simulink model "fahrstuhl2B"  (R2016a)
settings: Solver=ode45  StartTime=0.0  StopTime=Inf  FixedStep=1e-5  MaxStep=1e-4  RelTol=1e-3
undefined symbols (not defined in the file or in its folder): s0, tS, vF
libraries: simulink x3

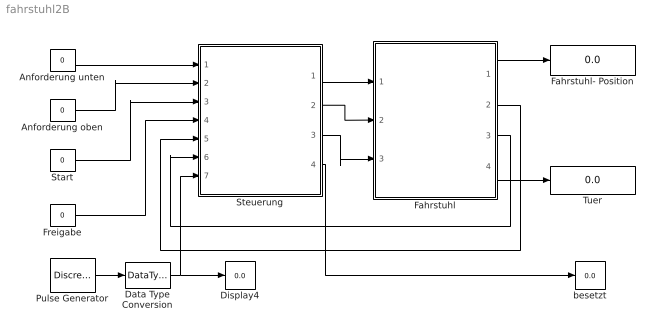
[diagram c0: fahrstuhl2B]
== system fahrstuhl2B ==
  Anforderung oben : Constant  Value=0  OutDataTypeStr=boolean
  Anforderung unten : Constant  Value=0  OutDataTypeStr=boolean
  Data Type Conversion : DataTypeConversion  OutDataTypeStr=boolean
  Display4 : Display
  Fahrstuhl : Subsystem
  Fahrstuhl- Position : Display
  Freigabe : Constant  Value=0  OutDataTypeStr=boolean
  Pulse Generator : DiscretePulseGenerator  PulseType=Time based  PulseWidth=50
  Start : Constant  Value=0  OutDataTypeStr=boolean
  Steuerung : Subsystem
  Tuer : Display
  besetzt : Display
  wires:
  Pulse Generator/1 -> Data Type Conversion/1
  Freigabe/1 -> Steuerung/4(F)
  Start/1 -> Steuerung/3(S)
  Anforderung oben/1 -> Steuerung/2(A2)
  Anforderung unten/1 -> Steuerung/1(A1)
  Fahrstuhl/1(z) -> Fahrstuhl- Position/1
  Steuerung/1(Mh) -> Fahrstuhl/1(Mh)
  Steuerung/2(Mr) -> Fahrstuhl/2(Mr)
  Steuerung/3(T) -> Fahrstuhl/3(Ti)
  Steuerung/4(Z) -> besetzt/1
  Fahrstuhl/4(T) -> Tuer/1
  Fahrstuhl/3(P2) -> Steuerung/6(P2)
  Fahrstuhl/2(P1) -> Steuerung/5(P1)
  Data Type Conversion/1 -> Steuerung/7(Takt), Display4/1

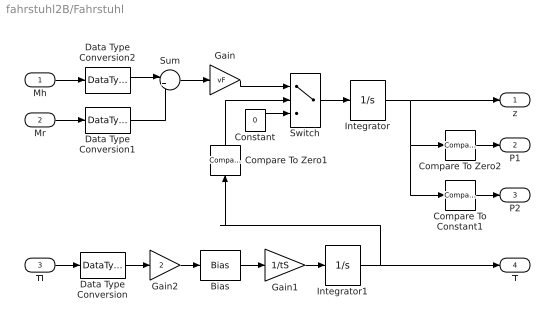
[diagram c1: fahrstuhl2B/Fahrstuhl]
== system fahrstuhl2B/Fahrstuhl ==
  Mh : Inport
  Mr : Inport  Port=2
  Ti : Inport  Port=3
  Bias : Bias  Bias=-1
  Compare To Constant1 : simulink/Logic and Bit Operations/Compare To Constant  SystemSampleTime=-1  relop===  const=1  LogicOutDataTypeMode=boolean
  Compare To Zero1 : simulink/Logic and Bit Operations/Compare To Zero  SystemSampleTime=-1  relop===  LogicOutDataTypeMode=uint8
  Compare To Zero2 : simulink/Logic and Bit Operations/Compare To Zero  SystemSampleTime=-1  relop===  LogicOutDataTypeMode=boolean
  Constant : Constant  Value=0
  Data Type Conversion : DataTypeConversion  OutDataTypeStr=double
  Data Type Conversion1 : DataTypeConversion  OutDataTypeStr=double
  Data Type Conversion2 : DataTypeConversion  OutDataTypeStr=double
  Gain : Gain  Gain=vF
  Gain1 : Gain  Gain=1/tS
  Gain2 : Gain  Gain=2
  Integrator : Integrator  LimitOutput=on  UpperSaturationLimit=1  LowerSaturationLimit=0
  Integrator1 : Integrator  LimitOutput=on  UpperSaturationLimit=1  LowerSaturationLimit=0
  Sum : Sum  Inputs=|+-
  Switch : Switch  Threshold=1
  z : Outport
  P1 : Outport  Port=2
  P2 : Outport  Port=3
  T : Outport  Port=4
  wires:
  Integrator/1 -> z/1, Compare To Constant1/1, Compare To Zero2/1
  Compare To Constant1/1 -> P2/1
  Compare To Zero2/1 -> P1/1
  Mh/1 -> Data Type Conversion2/1
  Mr/1 -> Data Type Conversion1/1
  Sum/1 -> Gain/1
  Gain1/1 -> Integrator1/1
  Integrator1/1 -> T/1, Compare To Zero1/1
  Gain2/1 -> Bias/1
  Bias/1 -> Gain1/1
  Ti/1 -> Data Type Conversion/1
  Gain/1 -> Switch/1
  Compare To Zero1/1 -> Switch/2
  Switch/1 -> Integrator/1
  Constant/1 -> Switch/3
  Data Type Conversion/1 -> Gain2/1
  Data Type Conversion1/1 -> Sum/2
  Data Type Conversion2/1 -> Sum/1

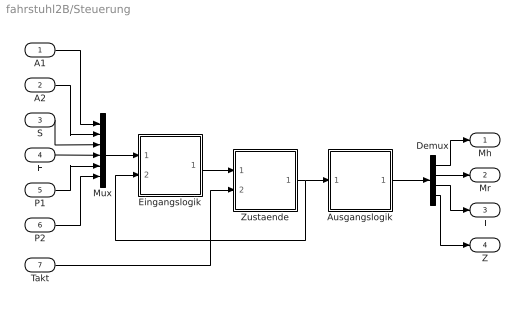
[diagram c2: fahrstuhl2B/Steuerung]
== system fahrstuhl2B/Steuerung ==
  A1 : Inport
  A2 : Inport  Port=2
  S : Inport  Port=3
  F : Inport  Port=4
  P1 : Inport  Port=5
  P2 : Inport  Port=6
  Takt : Inport  Port=7
  Ausgangslogik : Subsystem
  Demux : Demux
  Eingangslogik : Subsystem
  Mux : Mux  Inputs=6
  Zustaende : Subsystem
  Mh : Outport
  Mr : Outport  Port=2
  T : Outport  Port=3
  Z : Outport  Port=4
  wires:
  A1/1 -> Mux/1
  A2/1 -> Mux/2
  S/1 -> Mux/3
  F/1 -> Mux/4
  P1/1 -> Mux/5
  P2/1 -> Mux/6
  Demux/1 -> Mh/1
  Demux/2 -> Mr/1
  Demux/3 -> T/1
  Demux/4 -> Z/1
  Mux/1 -> Eingangslogik/1(E)
  Eingangslogik/1(A) -> Zustaende/1(D)
  Takt/1 -> Zustaende/2(CLK)
  Zustaende/1(Q) -> Ausgangslogik/1(E), Eingangslogik/2(Z)
  Ausgangslogik/1(A) -> Demux/1

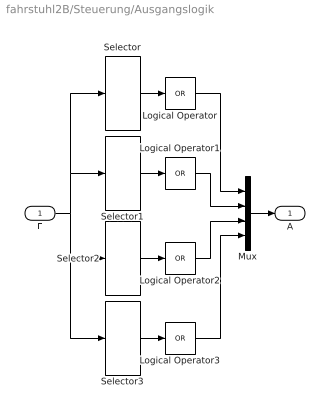
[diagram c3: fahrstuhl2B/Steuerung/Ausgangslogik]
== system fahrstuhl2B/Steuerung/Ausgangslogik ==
  E : Inport
  Logical Operator{,1..3} (4 alike) : Logic  Operator=OR  Inputs=1  AllPortsSameDT=off  OutDataTypeStr=boolean
  Mux : Mux
  Selector : Selector  InputPortWidth=10  IndexOptions=Index vector (dialog)  Indices=[3 10]  OutputSizes=1
  Selector1 : Selector  InputPortWidth=10  IndexOptions=Index vector (dialog)  Indices=[7 9]  OutputSizes=1
  Selector2 : Selector  InputPortWidth=10  IndexOptions=Index vector (dialog)  Indices=[2 4 6 8]  OutputSizes=1
  Selector3 : Selector  InputPortWidth=10  IndexOptions=Index vector (dialog)  Indices=[2 3 4 6 7 8 9 10]  OutputSizes=1
  A : Outport
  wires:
  Mux/1 -> A/1
  Logical Operator/1 -> Mux/1
  Selector/1 -> Logical Operator/1
  Selector1/1 -> Logical Operator1/1
  Logical Operator1/1 -> Mux/2
  Selector2/1 -> Logical Operator2/1
  Logical Operator2/1 -> Mux/3
  Selector3/1 -> Logical Operator3/1
  Logical Operator3/1 -> Mux/4
  E/1 -> Selector/1, Selector1/1, Selector2/1, Selector3/1

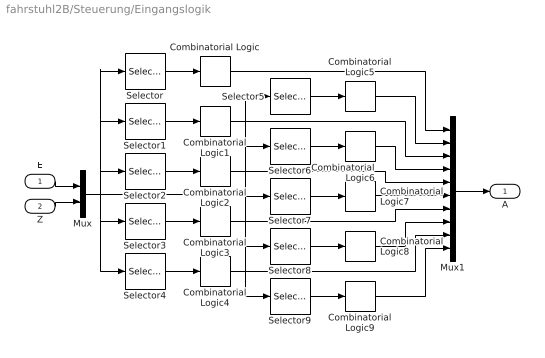
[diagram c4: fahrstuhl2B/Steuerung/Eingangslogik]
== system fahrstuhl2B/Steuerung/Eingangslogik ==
  E : Inport
  Z : Inport  Port=2
  Combinatorial Logic : CombinatorialLogic  TruthTable=[0;0;1;1;0;1;1;1;0;0;0;0;0;1;0;1;0;0;0;0;0;1;0;1;0;0;0;0;0;1;0;1]
  Combinatorial Logic{1,3..4,9} (4 alike) : CombinatorialLogic  TruthTable=[0;1;0;1;0;0;0;0;0;1;1;1;0;0;1;1]
  Combinatorial Logic2 : CombinatorialLogic  TruthTable=[0;1;0;1;0;1;1;1;0;0;0;0;0;0;1;1;0;0;0;0;0;0;1;1;0;0;0;0;0;0;1;1]
  Combinatorial Logic5 : CombinatorialLogic  TruthTable=[0;0;1;1;0;0;1;1;0;1;1;1;0;1;1;1;0;0;0;0;0;0;0;0;0;1;0;1;0;1;0;1;0;0;1;1;1;1;1;1;0;1;1;1;1;1;1;1;0;0;0;0;1;1;1;1;0;1;0;1;1;1;1;1]
  Combinatorial Logic6 : CombinatorialLogic  TruthTable=[0;1;0;1;0;1;1;1;0;0;0;0;0;0;1;1]
  Combinatorial Logic7 : CombinatorialLogic  TruthTable=[0;0;1;1;0;0;1;1;0;1;1;1;0;1;1;1;0;0;0;0;0;0;0;0;0;1;0;1;0;1;0;1;0;0;1;1;1;1;1;1;0;1;1;1;1;1;1;1;0;0;0;0;1;1;1;1;0;1;0;1;1;1;1;1]
  Combinatorial Logic8 : CombinatorialLogic  TruthTable=[0;1;0;1;0;1;1;1;0;0;0;0;0;0;1;1]
  Mux : Mux  Inputs=2
  Mux1 : Mux  Inputs=10
  Selector : Selector  InputPortWidth=16  IndexOptions=Index vector (dialog)  Indices=[1 2 4 7 14]  OutputSizes=1
  Selector1 : Selector  InputPortWidth=16  IndexOptions=Index vector (dialog)  Indices=[3 6 8 9]  OutputSizes=1
  Selector2 : Selector  InputPortWidth=16  IndexOptions=Index vector (dialog)  Indices=[1 2 4 10 11]  OutputSizes=1
  Selector3 : Selector  InputPortWidth=16  IndexOptions=Index vector (dialog)  Indices=[3 5 12 13]  OutputSizes=1
  Selector4 : Selector  InputPortWidth=16  IndexOptions=Index vector (dialog)  Indices=[1 5 11 15]  OutputSizes=1
  Selector5 : Selector  InputPortWidth=16  IndexOptions=Index vector (dialog)  Indices=[1 3 5 7 8 15]  OutputSizes=1
  Selector6 : Selector  InputPortWidth=16  IndexOptions=Index vector (dialog)  Indices=[4 6 9 10]  OutputSizes=1
  Selector7 : Selector  InputPortWidth=16  IndexOptions=Index vector (dialog)  Indices=[2 3 6 11 12 16]  OutputSizes=1
  Selector8 : Selector  InputPortWidth=16  IndexOptions=Index vector (dialog)  Indices=[4 5 13 14]  OutputSizes=1
  Selector9 : Selector  InputPortWidth=16  IndexOptions=Index vector (dialog)  Indices=[2 6 7 16]  OutputSizes=1
  A : Outport
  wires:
  E/1 -> Mux/1
  Z/1 -> Mux/2
  Selector/1 -> Combinatorial Logic/1
  Selector1/1 -> Combinatorial Logic1/1
  Selector2/1 -> Combinatorial Logic2/1
  Selector3/1 -> Combinatorial Logic3/1
  Selector4/1 -> Combinatorial Logic4/1
  Selector5/1 -> Combinatorial Logic5/1
  Selector6/1 -> Combinatorial Logic6/1
  Selector7/1 -> Combinatorial Logic7/1
  Selector8/1 -> Combinatorial Logic8/1
  Selector9/1 -> Combinatorial Logic9/1
  Mux1/1 -> A/1
  Combinatorial Logic/1 -> Mux1/1
  Combinatorial Logic5/1 -> Mux1/2
  Combinatorial Logic1/1 -> Mux1/3
  Combinatorial Logic6/1 -> Mux1/4
  Combinatorial Logic2/1 -> Mux1/5
  Combinatorial Logic7/1 -> Mux1/6
  Combinatorial Logic3/1 -> Mux1/7
  Combinatorial Logic8/1 -> Mux1/8
  Combinatorial Logic4/1 -> Mux1/9
  Combinatorial Logic9/1 -> Mux1/10
  Mux/1 -> Selector7/1, Selector5/1, Selector6/1, Selector9/1, Selector8/1, Selector/1, Selector1/1, Selector2/1, Selector4/1, Selector3/1

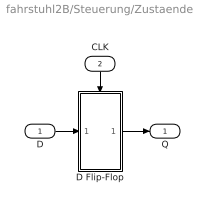
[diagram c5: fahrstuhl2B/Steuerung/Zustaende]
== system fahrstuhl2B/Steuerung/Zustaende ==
  D : Inport
  CLK : Inport  Port=2
  D Flip-Flop : Subsystem  TreatAsAtomicUnit=on
  Q : Outport  InitialOutput=0
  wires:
  D/1 -> D Flip-Flop/1(D)
  D Flip-Flop/1(Q) -> Q/1
  CLK/1 -> D Flip-Flop/Trigger

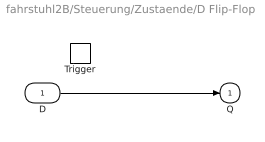
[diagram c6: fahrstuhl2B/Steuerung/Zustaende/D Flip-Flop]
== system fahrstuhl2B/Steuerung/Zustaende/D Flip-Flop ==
  D : Inport
  Trigger : TriggerPort  TriggerType=falling  VariantControl=Variant
  Q : Outport  InitialOutput=s0
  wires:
  D/1 -> Q/1
